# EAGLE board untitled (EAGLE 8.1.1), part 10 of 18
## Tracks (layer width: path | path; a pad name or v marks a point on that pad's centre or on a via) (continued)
S$9845 (continued)
  Bottom 0: 275.28,114.34 275.28,113.48
S$9846
  Bottom 0: 281.02,119.09 281.35,119.11
S$9847
  Bottom 0: 281.35,119.11 281.65,119.22
S$9848
  Bottom 0: 281.65,119.22 281.92,119.41
S$9849
  Bottom 0: 281.92,119.41 282.12,119.66
S$9850
  Bottom 0: 282.12,119.66 282.25,119.96
S$9851
  Bottom 0: 282.25,119.96 282.3,120.28
S$9852
  Bottom 0: 282.3,120.28 282.25,120.6
S$9853
  Bottom 0: 282.25,120.6 282.12,120.9
S$9854
  Bottom 0: 282.12,120.9 281.92,121.15
S$9855
  Bottom 0: 281.92,121.15 281.65,121.34
S$9856
  Bottom 0: 281.65,121.34 281.54,121.38
S$9857
  Bottom 0: 281.54,121.38 281.54,129.54
S$9858
  Bottom 0: 281.54,129.54 290.14,138.15
S$9859
  Bottom 0: 290.14,138.15 290.15,138.13
S$9860
  Bottom 0: 290.15,138.13 290.38,138.02
S$9861
  Bottom 0: 290.38,138.02 290.63,138
S$9862
  Bottom 0: 290.63,138 290.87,138.07
S$9863
  Bottom 0: 290.87,138.07 291.07,138.22
S$9864
  Bottom 0: 291.07,138.22 291.21,138.44
S$9865
  Bottom 0: 291.21,138.44 291.25,138.68
S$9866
  Bottom 0: 291.25,138.68 291.21,138.93
S$9867
  Bottom 0: 291.21,138.93 291.07,139.14
S$9868
  Bottom 0: 291.07,139.14 291,139.2
S$9869
  Bottom 0: 291,139.2 290.96,139.4
S$9870
  Bottom 0: 290.96,139.4 290.82,139.55
S$9871
  Bottom 0: 290.82,139.55 290.63,139.63
S$9872
  Bottom 0: 290.63,139.63 290.42,139.62
S$9873
  Bottom 0: 290.42,139.62 290.25,139.51
S$9874
  Bottom 0: 290.25,139.51 280.79,130.05
S$9875
  Bottom 0: 280.79,130.05 280.75,129.99
S$9876
  Bottom 0: 280.75,129.99 280.71,129.93
S$9877
  Bottom 0: 280.71,129.93 280.68,129.87
S$9878
  Bottom 0: 280.68,129.87 280.67,129.8
S$9879
  Bottom 0: 280.67,129.8 280.66,129.73
S$9880
  Bottom 0: 280.66,129.73 280.66,121.38
S$9881
  Bottom 0: 280.66,121.38 280.41,121.25
S$9882
  Bottom 0: 280.41,121.25 280.18,121.03
S$9883
  Bottom 0: 280.18,121.03 280,120.76
S$9884
  Bottom 0: 280,120.76 279.92,120.44
S$9885
  Bottom 0: 279.92,120.44 279.92,120.12
S$9886
  Bottom 0: 279.92,120.12 280,119.8
S$9887
  Bottom 0: 280,119.8 280.18,119.53
S$9888
  Bottom 0: 280.18,119.53 280.41,119.3
S$9889
  Bottom 0: 280.41,119.3 280.7,119.16
S$9890
  Bottom 0: 280.7,119.16 281.02,119.09
S$9891
  Bottom 0: 305.92,119.21 306.23,119.28
S$9892
  Bottom 0: 306.23,119.28 306.51,119.44
S$9893
  Bottom 0: 306.51,119.44 306.73,119.67
S$9894
  Bottom 0: 306.73,119.67 306.87,119.96
S$9895
  Bottom 0: 306.87,119.96 306.92,120.28
S$9896
  Bottom 0: 306.92,120.28 306.87,120.59
S$9897
  Bottom 0: 306.87,120.59 306.73,120.88
S$9898
  Bottom 0: 306.73,120.88 306.51,121.12
S$9899
  Bottom 0: 306.51,121.12 306.23,121.28
S$9900
  Bottom 0: 306.23,121.28 305.92,121.35
S$9901
  Bottom 0: 305.92,121.35 305.6,121.33
S$9902
  Bottom 0: 305.6,121.33 305.3,121.21
S$9903
  Bottom 0: 305.3,121.21 305.05,121.01
S$9904
  Bottom 0: 305.05,121.01 304.87,120.75
S$9905
  Bottom 0: 304.87,120.75 304.77,120.44
S$9906
  Bottom 0: 304.77,120.44 304.77,120.12
S$9907
  Bottom 0: 304.77,120.12 304.87,119.81
S$9908
  Bottom 0: 304.87,119.81 305.05,119.55
S$9909
  Bottom 0: 305.05,119.55 305.3,119.34
S$9910
  Bottom 0: 305.3,119.34 305.6,119.23
S$9911
  Bottom 0: 305.6,119.23 305.92,119.21
S$9912
  Bottom 0: 312.43,119.21 312.74,119.28
S$9913
  Bottom 0: 312.74,119.28 313.01,119.44
S$9914
  Bottom 0: 313.01,119.44 313.23,119.67
S$9915
  Bottom 0: 313.23,119.67 313.38,119.96
S$9916
  Bottom 0: 313.38,119.96 313.42,120.28
S$9917
  Bottom 0: 313.42,120.28 313.38,120.59
S$9918
  Bottom 0: 313.38,120.59 313.23,120.88
S$9919
  Bottom 0: 313.23,120.88 313.01,121.12
S$9920
  Bottom 0: 313.01,121.12 312.74,121.28
S$9921
  Bottom 0: 312.74,121.28 312.43,121.35
S$9922
  Bottom 0: 312.43,121.35 312.11,121.33
S$9923
  Bottom 0: 312.11,121.33 311.81,121.21
S$9924
  Bottom 0: 311.81,121.21 311.55,121.01
S$9925
  Bottom 0: 311.55,121.01 311.37,120.75
S$9926
  Bottom 0: 311.37,120.75 311.28,120.44
S$9927
  Bottom 0: 311.28,120.44 311.28,120.12
S$9928
  Bottom 0: 311.28,120.12 311.37,119.81
S$9929
  Bottom 0: 311.37,119.81 311.55,119.55
S$9930
  Bottom 0: 311.55,119.55 311.81,119.34
S$9931
  Bottom 0: 311.81,119.34 312.11,119.23
S$9932
  Bottom 0: 312.11,119.23 312.43,119.21
S$9933
  Bottom 0: 312.43,123.71 312.74,123.78
S$9934
  Bottom 0: 312.74,123.78 313.01,123.94
S$9935
  Bottom 0: 313.01,123.94 313.23,124.18
S$9936
  Bottom 0: 313.23,124.18 313.38,124.47
S$9937
  Bottom 0: 313.38,124.47 313.42,124.78
S$9938
  Bottom 0: 313.42,124.78 313.38,125.09
S$9939
  Bottom 0: 313.38,125.09 313.23,125.39
S$9940
  Bottom 0: 313.23,125.39 313.01,125.62
S$9941
  Bottom 0: 313.01,125.62 312.74,125.78
S$9942
  Bottom 0: 312.74,125.78 312.43,125.85
S$9943
  Bottom 0: 312.43,125.85 312.11,125.83
S$9944
  Bottom 0: 312.11,125.83 311.81,125.72
S$9945
  Bottom 0: 311.81,125.72 311.55,125.51
S$9946
  Bottom 0: 311.55,125.51 311.37,125.25
S$9947
  Bottom 0: 311.37,125.25 311.28,124.94
S$9948
  Bottom 0: 311.28,124.94 311.28,124.62
S$9949
  Bottom 0: 311.28,124.62 311.37,124.31
S$9950
  Bottom 0: 311.37,124.31 311.55,124.05
S$9951
  Bottom 0: 311.55,124.05 311.81,123.84
S$9952
  Bottom 0: 311.81,123.84 312.11,123.73
S$9953
  Bottom 0: 312.11,123.73 312.43,123.71
S$9954
  Bottom 0: 306.25,123.79 306.51,123.94
S$9955
  Bottom 0: 306.51,123.94 306.73,124.18
S$9956
  Bottom 0: 306.73,124.18 306.83,124.37
S$9957
  Bottom 0: 306.83,124.37 306.25,124.37
S$9958
  Bottom 0: 306.25,124.37 306.25,123.79
S$9959
  Bottom 0: 305.43,123.8 305.43,124.37
S$9960
  Bottom 0: 305.43,124.37 304.86,124.37
S$9961
  Bottom 0: 304.86,124.37 304.87,124.31
S$9962
  Bottom 0: 304.87,124.31 305.05,124.05
S$9963
  Bottom 0: 305.05,124.05 305.3,123.84
S$9964
  Bottom 0: 305.3,123.84 305.43,123.8
S$9965
  Bottom 0: 306.25,125.19 306.83,125.19
S$9966
  Bottom 0: 306.83,125.19 306.73,125.39
S$9967
  Bottom 0: 306.73,125.39 306.51,125.62
S$9968
  Bottom 0: 306.51,125.62 306.25,125.77
S$9969
  Bottom 0: 306.25,125.77 306.25,125.19
S$9970
  Bottom 0: 304.86,125.19 305.43,125.19
S$9971
  Bottom 0: 305.43,125.19 305.43,125.77
S$9972
  Bottom 0: 305.43,125.77 305.3,125.72
S$9973
  Bottom 0: 305.3,125.72 305.05,125.51
S$9974
  Bottom 0: 305.05,125.51 304.87,125.25
S$9975
  Bottom 0: 304.87,125.25 304.86,125.19
S$9976
  Bottom 0: 301.43,126.69 301.76,126.72
S$9977
  Bottom 0: 301.76,126.72 302.06,126.82
S$9978
  Bottom 0: 302.06,126.82 302.33,127.01
S$9979
  Bottom 0: 302.33,127.01 302.53,127.26
S$9980
  Bottom 0: 302.53,127.26 302.66,127.56
S$9981
  Bottom 0: 302.66,127.56 302.71,127.88
S$9982
  Bottom 0: 302.71,127.88 302.66,128.2
S$9983
  Bottom 0: 302.66,128.2 302.53,128.5
S$9984
  Bottom 0: 302.53,128.5 302.33,128.76
S$9985
  Bottom 0: 302.33,128.76 302.06,128.95
S$9986
  Bottom 0: 302.06,128.95 301.76,129.05
S$9987
  Bottom 0: 301.76,129.05 301.43,129.07
S$9988
  Bottom 0: 301.43,129.07 301.11,129.01
S$9989
  Bottom 0: 301.11,129.01 300.82,128.86
S$9990
  Bottom 0: 300.82,128.86 300.59,128.64
S$9991
  Bottom 0: 300.59,128.64 300.42,128.36
S$9992
  Bottom 0: 300.42,128.36 300.33,128.05
S$9993
  Bottom 0: 300.33,128.05 300.33,127.72
S$9994
  Bottom 0: 300.33,127.72 300.42,127.41
S$9995
  Bottom 0: 300.42,127.41 300.59,127.13
S$9996
  Bottom 0: 300.59,127.13 300.82,126.91
S$9997
  Bottom 0: 300.82,126.91 301.11,126.76
S$9998
  Bottom 0: 301.11,126.76 301.43,126.69
S$9999
  Bottom 0: 303.97,126.69 304.3,126.72
S$10000
  Bottom 0: 304.3,126.72 304.6,126.82
S$10001
  Bottom 0: 304.6,126.82 304.87,127.01
S$10002
  Bottom 0: 304.87,127.01 305.07,127.26
S$10003
  Bottom 0: 305.07,127.26 305.2,127.56
S$10004
  Bottom 0: 305.2,127.56 305.25,127.88
S$10005
  Bottom 0: 305.25,127.88 305.2,128.2
S$10006
  Bottom 0: 305.2,128.2 305.07,128.5
S$10007
  Bottom 0: 305.07,128.5 304.87,128.76
S$10008
  Bottom 0: 304.87,128.76 304.6,128.95
S$10009
  Bottom 0: 304.6,128.95 304.3,129.05
S$10010
  Bottom 0: 304.3,129.05 303.97,129.07
S$10011
  Bottom 0: 303.97,129.07 303.65,129.01
S$10012
  Bottom 0: 303.65,129.01 303.36,128.86
S$10013
  Bottom 0: 303.36,128.86 303.13,128.64
S$10014
  Bottom 0: 303.13,128.64 302.96,128.36
S$10015
  Bottom 0: 302.96,128.36 302.87,128.05
S$10016
  Bottom 0: 302.87,128.05 302.87,127.72
S$10017
  Bottom 0: 302.87,127.72 302.96,127.41
S$10018
  Bottom 0: 302.96,127.41 303.13,127.13
S$10019
  Bottom 0: 303.13,127.13 303.36,126.91
S$10020
  Bottom 0: 303.36,126.91 303.65,126.76
S$10021
  Bottom 0: 303.65,126.76 303.97,126.69
S$10022
  Bottom 0: 309.05,126.69 309.38,126.72
S$10023
  Bottom 0: 309.38,126.72 309.68,126.82
S$10024
  Bottom 0: 309.68,126.82 309.95,127.01
S$10025
  Bottom 0: 309.95,127.01 310.15,127.26
S$10026
  Bottom 0: 310.15,127.26 310.28,127.56
S$10027
  Bottom 0: 310.28,127.56 310.33,127.88
S$10028
  Bottom 0: 310.33,127.88 310.28,128.2
S$10029
  Bottom 0: 310.28,128.2 310.15,128.5
S$10030
  Bottom 0: 310.15,128.5 309.95,128.76
S$10031
  Bottom 0: 309.95,128.76 309.68,128.95
S$10032
  Bottom 0: 309.68,128.95 309.38,129.05
S$10033
  Bottom 0: 309.38,129.05 309.05,129.07
S$10034
  Bottom 0: 309.05,129.07 308.73,129.01
S$10035
  Bottom 0: 308.73,129.01 308.44,128.86
S$10036
  Bottom 0: 308.44,128.86 308.21,128.64
S$10037
  Bottom 0: 308.21,128.64 308.04,128.36
S$10038
  Bottom 0: 308.04,128.36 307.95,128.05
S$10039
  Bottom 0: 307.95,128.05 307.95,127.72
S$10040
  Bottom 0: 307.95,127.72 308.04,127.41
S$10041
  Bottom 0: 308.04,127.41 308.21,127.13
S$10042
  Bottom 0: 308.21,127.13 308.44,126.91
S$10043
  Bottom 0: 308.44,126.91 308.73,126.76
S$10044
  Bottom 0: 308.73,126.76 309.05,126.69
S$10045
  Bottom 0: 289.28,126.79 289.36,126.82
S$10046
  Bottom 0: 289.36,126.82 289.63,127.01
S$10047
  Bottom 0: 289.63,127.01 289.83,127.26
S$10048
  Bottom 0: 289.83,127.26 289.9,127.42
S$10049
  Bottom 0: 289.9,127.42 289.28,127.42
S$10050
  Bottom 0: 289.28,127.42 289.28,126.79
S$10051
  Bottom 0: 288.35,126.8 288.35,127.42
S$10052
  Bottom 0: 288.35,127.42 287.71,127.42
S$10053
  Bottom 0: 287.71,127.42 287.72,127.41
S$10054
  Bottom 0: 287.72,127.41 287.89,127.13
S$10055
  Bottom 0: 287.89,127.13 288.12,126.91
S$10056
  Bottom 0: 288.12,126.91 288.35,126.8
S$10057
  Bottom 0: 289.28,128.35 289.9,128.35
S$10058
  Bottom 0: 289.9,128.35 289.83,128.5
S$10059
  Bottom 0: 289.83,128.5 289.63,128.76
S$10060
  Bottom 0: 289.63,128.76 289.36,128.95
S$10061
  Bottom 0: 289.36,128.95 289.28,128.98
S$10062
  Bottom 0: 289.28,128.98 289.28,128.35
S$10063
  Bottom 0: 287.71,128.35 288.35,128.35
S$10064
  Bottom 0: 288.35,128.35 288.35,128.97
S$10065
  Bottom 0: 288.35,128.97 288.12,128.86
S$10066
  Bottom 0: 288.12,128.86 287.89,128.64
S$10067
  Bottom 0: 287.89,128.64 287.72,128.36
S$10068
  Bottom 0: 287.72,128.36 287.71,128.35
S$10069
  Bottom 0: 292.49,130.78 292.73,130.85
S$10070
  Bottom 0: 292.73,130.85 292.93,131
S$10071
  Bottom 0: 292.93,131 293.06,131.21
S$10072
  Bottom 0: 293.06,131.21 293.11,131.46
S$10073
  Bottom 0: 293.11,131.46 293.06,131.71
S$10074
  Bottom 0: 293.06,131.71 292.93,131.92
S$10075
  Bottom 0: 292.93,131.92 292.86,131.97
S$10076
  Bottom 0: 292.86,131.97 292.86,133.85
S$10077
  Bottom 0: 292.86,133.85 301.05,142.03
S$10078
  Bottom 0: 301.05,142.03 301.11,142
S$10079
  Bottom 0: 301.11,142 301.43,141.93
S$10080
  Bottom 0: 301.43,141.93 301.76,141.96
S$10081
  Bottom 0: 301.76,141.96 302.06,142.06
S$10082
  Bottom 0: 302.06,142.06 302.33,142.25
S$10083
  Bottom 0: 302.33,142.25 302.53,142.5
S$10084
  Bottom 0: 302.53,142.5 302.66,142.8
S$10085
  Bottom 0: 302.66,142.8 302.71,143.12
S$10086
  Bottom 0: 302.71,143.12 302.66,143.44
S$10087
  Bottom 0: 302.66,143.44 302.53,143.74
S$10088
  Bottom 0: 302.53,143.74 302.33,144
S$10089
  Bottom 0: 302.33,144 302.06,144.19
S$10090
  Bottom 0: 302.06,144.19 301.76,144.29
S$10091
  Bottom 0: 301.76,144.29 301.43,144.31
S$10092
  Bottom 0: 301.43,144.31 301.11,144.25
S$10093
  Bottom 0: 301.11,144.25 300.82,144.1
S$10094
  Bottom 0: 300.82,144.1 300.59,143.88
S$10095
  Bottom 0: 300.59,143.88 300.42,143.6
S$10096
  Bottom 0: 300.42,143.6 300.33,143.29
S$10097
  Bottom 0: 300.33,143.29 300.33,142.96
S$10098
  Bottom 0: 300.33,142.96 300.42,142.66
S$10099
  Bottom 0: 300.42,142.66 292.11,134.35
S$10100
  Bottom 0: 292.11,134.35 292.02,134.24
S$10101
  Bottom 0: 292.02,134.24 292,134.17
S$10102
  Bottom 0: 292,134.17 291.98,134.11
S$10103
  Bottom 0: 291.98,134.11 291.98,134.04
S$10104
  Bottom 0: 291.98,134.04 291.98,131.97
S$10105
  Bottom 0: 291.98,131.97 291.84,131.82
S$10106
  Bottom 0: 291.84,131.82 291.75,131.59
S$10107
  Bottom 0: 291.75,131.59 291.75,131.33
S$10108
  Bottom 0: 291.75,131.33 291.84,131.1
S$10109
  Bottom 0: 291.84,131.1 292.01,130.91
S$10110
  Bottom 0: 292.01,130.91 292.24,130.8
S$10111
  Bottom 0: 292.24,130.8 292.49,130.78
S$10112
  Bottom 0: 311.59,141.93 311.92,141.96
S$10113
  Bottom 0: 311.92,141.96 312.22,142.06
S$10114
  Bottom 0: 312.22,142.06 312.49,142.25
S$10115
  Bottom 0: 312.49,142.25 312.69,142.5
S$10116
  Bottom 0: 312.69,142.5 312.82,142.8
S$10117
  Bottom 0: 312.82,142.8 312.87,143.12
S$10118
  Bottom 0: 312.87,143.12 312.82,143.44
S$10119
  Bottom 0: 312.82,143.44 312.69,143.74
S$10120
  Bottom 0: 312.69,143.74 312.49,144
S$10121
  Bottom 0: 312.49,144 312.22,144.19
S$10122
  Bottom 0: 312.22,144.19 311.92,144.29
S$10123
  Bottom 0: 311.92,144.29 311.59,144.31
S$10124
  Bottom 0: 311.59,144.31 311.27,144.25
S$10125
  Bottom 0: 311.27,144.25 310.98,144.1
S$10126
  Bottom 0: 310.98,144.1 310.75,143.88
S$10127
  Bottom 0: 310.75,143.88 310.58,143.6
S$10128
  Bottom 0: 310.58,143.6 310.49,143.29
S$10129
  Bottom 0: 310.49,143.29 310.49,142.96
S$10130
  Bottom 0: 310.49,142.96 310.58,142.65
S$10131
  Bottom 0: 310.58,142.65 310.75,142.37
S$10132
  Bottom 0: 310.75,142.37 310.98,142.15
S$10133
  Bottom 0: 310.98,142.15 311.27,142
S$10134
  Bottom 0: 311.27,142 311.59,141.93
S$10135
  Bottom 0: 309.05,141.93 309.38,141.96
S$10136
  Bottom 0: 309.38,141.96 309.68,142.06
S$10137
  Bottom 0: 309.68,142.06 309.95,142.25
S$10138
  Bottom 0: 309.95,142.25 310.15,142.5
S$10139
  Bottom 0: 310.15,142.5 310.28,142.8
S$10140
  Bottom 0: 310.28,142.8 310.33,143.12
S$10141
  Bottom 0: 310.33,143.12 310.28,143.44
S$10142
  Bottom 0: 310.28,143.44 310.15,143.74
S$10143
  Bottom 0: 310.15,143.74 309.95,144
S$10144
  Bottom 0: 309.95,144 309.68,144.19
S$10145
  Bottom 0: 309.68,144.19 309.38,144.29
S$10146
  Bottom 0: 309.38,144.29 309.05,144.31
S$10147
  Bottom 0: 309.05,144.31 308.73,144.25
S$10148
  Bottom 0: 308.73,144.25 308.44,144.1
S$10149
  Bottom 0: 308.44,144.1 308.21,143.88
S$10150
  Bottom 0: 308.21,143.88 308.04,143.6
S$10151
  Bottom 0: 308.04,143.6 307.95,143.29
S$10152
  Bottom 0: 307.95,143.29 307.95,142.96
S$10153
  Bottom 0: 307.95,142.96 308.04,142.65
S$10154
  Bottom 0: 308.04,142.65 308.21,142.37
S$10155
  Bottom 0: 308.21,142.37 308.44,142.15
S$10156
  Bottom 0: 308.44,142.15 308.73,142
S$10157
  Bottom 0: 308.73,142 309.05,141.93
S$10158
  Bottom 0: 298.89,141.93 299.22,141.96
S$10159
  Bottom 0: 299.22,141.96 299.52,142.06
S$10160
  Bottom 0: 299.52,142.06 299.79,142.25
S$10161
  Bottom 0: 299.79,142.25 299.99,142.5
S$10162
  Bottom 0: 299.99,142.5 300.12,142.8
S$10163
  Bottom 0: 300.12,142.8 300.17,143.12
S$10164
  Bottom 0: 300.17,143.12 300.12,143.44
S$10165
  Bottom 0: 300.12,143.44 300.06,143.58
S$10166
  Bottom 0: 300.06,143.58 301.1,144.63
S$10167
  Bottom 0: 301.1,144.63 301.14,144.68
S$10168
  Bottom 0: 301.14,144.68 301.18,144.74
S$10169
  Bottom 0: 301.18,144.74 301.2,144.8
S$10170
  Bottom 0: 301.2,144.8 301.22,144.86
S$10171
  Bottom 0: 301.22,144.86 301.22,144.94
S$10172
  Bottom 0: 301.22,144.94 301.22,150.65
S$10173
  Bottom 0: 301.22,150.65 301.28,150.63
S$10174
  Bottom 0: 301.28,150.63 301.63,150.61
S$10175
  Bottom 0: 301.63,150.61 301.98,150.67
S$10176
  Bottom 0: 301.98,150.67 302.29,150.82
S$10177
  Bottom 0: 302.29,150.82 302.56,151.05
S$10178
  Bottom 0: 302.56,151.05 302.77,151.33
S$10179
  Bottom 0: 302.77,151.33 302.89,151.66
S$10180
  Bottom 0: 302.89,151.66 302.94,152
S$10181
  Bottom 0: 302.94,152 302.89,152.35
S$10182
  Bottom 0: 302.89,152.35 302.77,152.67
S$10183
  Bottom 0: 302.77,152.67 302.56,152.96
S$10184
  Bottom 0: 302.56,152.96 302.29,153.18
S$10185
  Bottom 0: 302.29,153.18 301.98,153.34
S$10186
  Bottom 0: 301.98,153.34 301.63,153.39
S$10187
  Bottom 0: 301.63,153.39 301.28,153.38
S$10188
  Bottom 0: 301.28,153.38 301.17,153.34
S$10189
  Bottom 0: 301.17,153.34 300.87,153.39
S$10190
  Bottom 0: 300.87,153.39 300.52,153.38
S$10191
  Bottom 0: 300.52,153.38 300.19,153.27
S$10192
  Bottom 0: 300.19,153.27 299.89,153.08
S$10193
  Bottom 0: 299.89,153.08 299.65,152.83
S$10194
  Bottom 0: 299.65,152.83 299.48,152.52
S$10195
  Bottom 0: 299.48,152.52 299.39,152.18
S$10196
  Bottom 0: 299.39,152.18 299.39,151.83
S$10197
  Bottom 0: 299.39,151.83 299.48,151.49
S$10198
  Bottom 0: 299.48,151.49 299.65,151.18
S$10199
  Bottom 0: 299.65,151.18 299.89,150.93
S$10200
  Bottom 0: 299.89,150.93 300.19,150.74
S$10201
  Bottom 0: 300.19,150.74 300.34,150.69
S$10202
  Bottom 0: 300.34,150.69 300.34,145.12
S$10203
  Bottom 0: 300.34,145.12 299.44,144.22
S$10204
  Bottom 0: 299.44,144.22 299.22,144.29
S$10205
  Bottom 0: 299.22,144.29 298.89,144.31
S$10206
  Bottom 0: 298.89,144.31 298.57,144.25
S$10207
  Bottom 0: 298.57,144.25 298.28,144.1
S$10208
  Bottom 0: 298.28,144.1 298.05,143.88
S$10209
  Bottom 0: 298.05,143.88 297.88,143.6
S$10210
  Bottom 0: 297.88,143.6 297.79,143.29
S$10211
  Bottom 0: 297.79,143.29 297.79,142.96
S$10212
  Bottom 0: 297.79,142.96 297.88,142.65
S$10213
  Bottom 0: 297.88,142.65 298.05,142.37
S$10214
  Bottom 0: 298.05,142.37 298.28,142.15
S$10215
  Bottom 0: 298.28,142.15 298.57,142
S$10216
  Bottom 0: 298.57,142 298.89,141.93
S$10217
  Bottom 0: 296.35,141.93 296.68,141.96
S$10218
  Bottom 0: 296.68,141.96 296.98,142.06
S$10219
  Bottom 0: 296.98,142.06 297.25,142.25
S$10220
  Bottom 0: 297.25,142.25 297.45,142.5
S$10221
  Bottom 0: 297.45,142.5 297.58,142.8
S$10222
  Bottom 0: 297.58,142.8 297.63,143.12
S$10223
  Bottom 0: 297.63,143.12 297.58,143.44
S$10224
  Bottom 0: 297.58,143.44 297.45,143.74
S$10225
  Bottom 0: 297.45,143.74 297.25,144
S$10226
  Bottom 0: 297.25,144 296.98,144.19
S$10227
  Bottom 0: 296.98,144.19 296.68,144.29
S$10228
  Bottom 0: 296.68,144.29 296.35,144.31
S$10229
  Bottom 0: 296.35,144.31 296.03,144.25
S$10230
  Bottom 0: 296.03,144.25 295.74,144.1
S$10231
  Bottom 0: 295.74,144.1 295.51,143.88
S$10232
  Bottom 0: 295.51,143.88 295.34,143.6
S$10233
  Bottom 0: 295.34,143.6 295.25,143.29
S$10234
  Bottom 0: 295.25,143.29 295.25,142.96
S$10235
  Bottom 0: 295.25,142.96 295.34,142.65
S$10236
  Bottom 0: 295.34,142.65 295.51,142.37
S$10237
  Bottom 0: 295.51,142.37 295.74,142.15
S$10238
  Bottom 0: 295.74,142.15 296.03,142
S$10239
  Bottom 0: 296.03,142 296.35,141.93
S$10240
  Bottom 0: 288.73,141.93 289.06,141.96
S$10241
  Bottom 0: 289.06,141.96 289.36,142.06
S$10242
  Bottom 0: 289.36,142.06 289.63,142.25
S$10243
  Bottom 0: 289.63,142.25 289.83,142.5
S$10244
  Bottom 0: 289.83,142.5 289.96,142.8
S$10245
  Bottom 0: 289.96,142.8 290.01,143.12
S$10246
  Bottom 0: 290.01,143.12 289.96,143.44
S$10247
  Bottom 0: 289.96,143.44 289.83,143.74
S$10248
  Bottom 0: 289.83,143.74 289.63,144
S$10249
  Bottom 0: 289.63,144 289.36,144.19
S$10250
  Bottom 0: 289.36,144.19 289.06,144.29
S$10251
  Bottom 0: 289.06,144.29 288.73,144.31
S$10252
  Bottom 0: 288.73,144.31 288.41,144.25
S$10253
  Bottom 0: 288.41,144.25 288.12,144.1
S$10254
  Bottom 0: 288.12,144.1 287.89,143.88
S$10255
  Bottom 0: 287.89,143.88 287.72,143.6
S$10256
  Bottom 0: 287.72,143.6 287.63,143.29
S$10257
  Bottom 0: 287.63,143.29 287.63,142.96
S$10258
  Bottom 0: 287.63,142.96 287.72,142.65
S$10259
  Bottom 0: 287.72,142.65 287.89,142.37
S$10260
  Bottom 0: 287.89,142.37 288.12,142.15
S$10261
  Bottom 0: 288.12,142.15 288.41,142
S$10262
  Bottom 0: 288.41,142 288.73,141.93
S$10263
  Bottom 0: 286.19,141.93 286.52,141.96
S$10264
  Bottom 0: 286.52,141.96 286.82,142.06
S$10265
  Bottom 0: 286.82,142.06 287.09,142.25
S$10266
  Bottom 0: 287.09,142.25 287.29,142.5
S$10267
  Bottom 0: 287.29,142.5 287.42,142.8
S$10268
  Bottom 0: 287.42,142.8 287.47,143.12
S$10269
  Bottom 0: 287.47,143.12 287.42,143.44
S$10270
  Bottom 0: 287.42,143.44 287.29,143.74
S$10271
  Bottom 0: 287.29,143.74 287.09,144
S$10272
  Bottom 0: 287.09,144 286.82,144.19
S$10273
  Bottom 0: 286.82,144.19 286.52,144.29
S$10274
  Bottom 0: 286.52,144.29 286.19,144.31
S$10275
  Bottom 0: 286.19,144.31 285.87,144.25
S$10276
  Bottom 0: 285.87,144.25 285.58,144.1
S$10277
  Bottom 0: 285.58,144.1 285.35,143.88
S$10278
  Bottom 0: 285.35,143.88 285.18,143.6
S$10279
  Bottom 0: 285.18,143.6 285.09,143.29
S$10280
  Bottom 0: 285.09,143.29 285.09,142.96
S$10281
  Bottom 0: 285.09,142.96 285.18,142.65
S$10282
  Bottom 0: 285.18,142.65 285.35,142.37
S$10283
  Bottom 0: 285.35,142.37 285.58,142.15
S$10284
  Bottom 0: 285.58,142.15 285.87,142
S$10285
  Bottom 0: 285.87,142 286.19,141.93
S$10286
  Bottom 0: 294.36,142.03 294.44,142.06
S$10287
  Bottom 0: 294.44,142.06 294.71,142.25
S$10288
  Bottom 0: 294.71,142.25 294.91,142.5
S$10289
  Bottom 0: 294.91,142.5 294.98,142.66
S$10290
  Bottom 0: 294.98,142.66 294.36,142.66
S$10291
  Bottom 0: 294.36,142.66 294.36,142.03
S$10292
  Bottom 0: 291.82,142.03 291.9,142.06
S$10293
  Bottom 0: 291.9,142.06 292.17,142.25
S$10294
  Bottom 0: 292.17,142.25 292.37,142.5
S$10295
  Bottom 0: 292.37,142.5 292.44,142.66
S$10296
  Bottom 0: 292.44,142.66 291.82,142.66
S$10297
  Bottom 0: 291.82,142.66 291.82,142.03
S$10298
  Bottom 0: 293.43,142.04 293.43,142.66
S$10299
  Bottom 0: 293.43,142.66 292.79,142.66
S$10300
  Bottom 0: 292.79,142.66 292.8,142.65
S$10301
  Bottom 0: 292.8,142.65 292.97,142.37
S$10302
  Bottom 0: 292.97,142.37 293.2,142.15
S$10303
  Bottom 0: 293.2,142.15 293.43,142.04
S$10304
  Bottom 0: 290.89,142.04 290.89,142.66
S$10305
  Bottom 0: 290.89,142.66 290.25,142.66
S$10306
  Bottom 0: 290.25,142.66 290.26,142.65
S$10307
  Bottom 0: 290.26,142.65 290.43,142.37
S$10308
  Bottom 0: 290.43,142.37 290.66,142.15
S$10309
  Bottom 0: 290.66,142.15 290.89,142.04
S$10310
  Bottom 0: 294.36,143.59 294.98,143.59
S$10311
  Bottom 0: 294.98,143.59 294.91,143.74
S$10312
  Bottom 0: 294.91,143.74 294.71,144
S$10313
  Bottom 0: 294.71,144 294.44,144.19
S$10314
  Bottom 0: 294.44,144.19 294.36,144.22
S$10315
  Bottom 0: 294.36,144.22 294.36,143.59
S$10316
  Bottom 0: 292.79,143.59 293.43,143.59
S$10317
  Bottom 0: 293.43,143.59 293.43,144.21
S$10318
  Bottom 0: 293.43,144.21 293.2,144.1
S$10319
  Bottom 0: 293.2,144.1 292.97,143.88
S$10320
  Bottom 0: 292.97,143.88 292.8,143.6
S$10321
  Bottom 0: 292.8,143.6 292.79,143.59
S$10322
  Bottom 0: 291.82,143.59 292.44,143.59
S$10323
  Bottom 0: 292.44,143.59 292.37,143.74
S$10324
  Bottom 0: 292.37,143.74 292.17,144
S$10325
  Bottom 0: 292.17,144 291.9,144.19
S$10326
  Bottom 0: 291.9,144.19 291.82,144.22
S$10327
  Bottom 0: 291.82,144.22 291.82,143.59
S$10328
  Bottom 0: 290.25,143.59 290.89,143.59
S$10329
  Bottom 0: 290.89,143.59 290.89,144.21
S$10330
  Bottom 0: 290.89,144.21 290.66,144.1
S$10331
  Bottom 0: 290.66,144.1 290.43,143.88
S$10332
  Bottom 0: 290.43,143.88 290.26,143.6
S$10333
  Bottom 0: 290.26,143.6 290.25,143.59
S$10334
  Bottom 0: 294.52,148.07 294.82,148.13
S$10335
  Bottom 0: 294.82,148.13 294.93,148.09
S$10336
  Bottom 0: 294.93,148.09 295.28,148.07
S$10337
  Bottom 0: 295.28,148.07 295.63,148.13
S$10338
  Bottom 0: 295.63,148.13 295.94,148.28
S$10339
  Bottom 0: 295.94,148.28 296.21,148.51
S$10340
  Bottom 0: 296.21,148.51 296.42,148.79
S$10341
  Bottom 0: 296.42,148.79 296.55,149.12
S$10342
  Bottom 0: 296.55,149.12 296.59,149.46
S$10343
  Bottom 0: 296.59,149.46 296.55,149.81
S$10344
  Bottom 0: 296.55,149.81 296.42,150.13
S$10345
  Bottom 0: 296.42,150.13 296.21,150.42
S$10346
  Bottom 0: 296.21,150.42 295.94,150.64
S$10347
  Bottom 0: 295.94,150.64 295.63,150.79
S$10348
  Bottom 0: 295.63,150.79 295.28,150.85
S$10349
  Bottom 0: 295.28,150.85 294.93,150.84
S$10350
  Bottom 0: 294.93,150.84 294.82,150.8
S$10351
  Bottom 0: 294.82,150.8 294.52,150.85
S$10352
  Bottom 0: 294.52,150.85 294.17,150.84
S$10353
  Bottom 0: 294.17,150.84 293.83,150.73
S$10354
  Bottom 0: 293.83,150.73 293.54,150.54
S$10355
  Bottom 0: 293.54,150.54 293.3,150.29
S$10356
  Bottom 0: 293.3,150.29 293.13,149.98
S$10357
  Bottom 0: 293.13,149.98 293.11,149.91
S$10358
  Bottom 0: 293.11,149.91 289.96,149.91
S$10359
  Bottom 0: 289.96,149.91 289.21,150.66
S$10360
  Bottom 0: 289.21,150.66 289.23,150.68
S$10361
  Bottom 0: 289.23,150.68 289.27,150.98
S$10362
  Bottom 0: 289.27,150.98 289.23,151.28
S$10363
  Bottom 0: 289.23,151.28 289.09,151.56
S$10364
  Bottom 0: 289.09,151.56 288.89,151.78
S$10365
  Bottom 0: 288.89,151.78 288.62,151.93
S$10366
  Bottom 0: 288.62,151.93 288.33,151.99
S$10367
  Bottom 0: 288.33,151.99 288.03,151.97
S$10368
  Bottom 0: 288.03,151.97 287.74,151.86
S$10369
  Bottom 0: 287.74,151.86 287.51,151.67
S$10370
  Bottom 0: 287.51,151.67 287.34,151.43
S$10371
  Bottom 0: 287.34,151.43 287.25,151.13
S$10372
  Bottom 0: 287.25,151.13 287.25,150.83
S$10373
  Bottom 0: 287.25,150.83 287.34,150.54
S$10374
  Bottom 0: 287.34,150.54 287.51,150.29
S$10375
  Bottom 0: 287.51,150.29 287.74,150.1
S$10376
  Bottom 0: 287.74,150.1 288.03,149.99
S$10377
  Bottom 0: 288.03,149.99 288.33,149.97
S$10378
  Bottom 0: 288.33,149.97 288.58,150.03
S$10379
  Bottom 0: 288.58,150.03 289.46,149.15
S$10380
  Bottom 0: 289.46,149.15 289.51,149.11
S$10381
  Bottom 0: 289.51,149.11 289.57,149.07
S$10382
  Bottom 0: 289.57,149.07 289.64,149.04
S$10383
  Bottom 0: 289.64,149.04 289.7,149.03
S$10384
  Bottom 0: 289.7,149.03 289.77,149.02
S$10385
  Bottom 0: 289.77,149.02 293.11,149.02
S$10386
  Bottom 0: 293.11,149.02 293.13,148.95
S$10387
  Bottom 0: 293.13,148.95 293.3,148.64
S$10388
  Bottom 0: 293.3,148.64 293.54,148.39
S$10389
  Bottom 0: 293.54,148.39 293.83,148.2
S$10390
  Bottom 0: 293.83,148.2 294.17,148.09
S$10391
  Bottom 0: 294.17,148.09 294.52,148.07
S$10392
  Bottom 0: 296.97,152.26 297.35,152.3
S$10393
  Bottom 0: 297.35,152.3 297.73,152.26
S$10394
  Bottom 0: 297.73,152.26 298.18,152.3
S$10395
  Bottom 0: 298.18,152.3 298.61,152.43
S$10396
  Bottom 0: 298.61,152.43 299,152.64
S$10397
  Bottom 0: 299,152.64 299.35,152.93
S$10398
  Bottom 0: 299.35,152.93 299.63,153.27
S$10399
  Bottom 0: 299.63,153.27 299.85,153.67
S$10400
  Bottom 0: 299.85,153.67 299.97,154.1
S$10401
  Bottom 0: 299.97,154.1 300.02,154.54
S$10402
  Bottom 0: 300.02,154.54 299.97,154.99
S$10403
  Bottom 0: 299.97,154.99 299.85,155.42
S$10404
  Bottom 0: 299.85,155.42 299.63,155.81
S$10405
  Bottom 0: 299.63,155.81 299.35,156.16
S$10406
  Bottom 0: 299.35,156.16 299,156.44
S$10407
  Bottom 0: 299,156.44 298.61,156.66
S$10408
  Bottom 0: 298.61,156.66 298.18,156.78
S$10409
  Bottom 0: 298.18,156.78 297.73,156.83
S$10410
  Bottom 0: 297.73,156.83 297.35,156.79
S$10411
  Bottom 0: 297.35,156.79 296.97,156.83
S$10412
  Bottom 0: 296.97,156.83 296.52,156.78
S$10413
  Bottom 0: 296.52,156.78 296.1,156.66
S$10414
  Bottom 0: 296.1,156.66 295.7,156.44
S$10415
  Bottom 0: 295.7,156.44 295.36,156.16
S$10416
  Bottom 0: 295.36,156.16 295.07,155.81
S$10417
  Bottom 0: 295.07,155.81 294.86,155.42
S$10418
  Bottom 0: 294.86,155.42 294.73,154.99
S$10419
  Bottom 0: 294.73,154.99 294.69,154.54
S$10420
  Bottom 0: 294.69,154.54 294.73,154.1
S$10421
  Bottom 0: 294.73,154.1 294.86,153.67
S$10422
  Bottom 0: 294.86,153.67 295.07,153.27
S$10423
  Bottom 0: 295.07,153.27 295.36,152.93
S$10424
  Bottom 0: 295.36,152.93 295.7,152.64
S$10425
  Bottom 0: 295.7,152.64 296.1,152.43
S$10426
  Bottom 0: 296.1,152.43 296.52,152.3
S$10427
  Bottom 0: 296.52,152.3 296.97,152.26
S$10428
  Bottom 0: 288.33,157.59 288.62,157.66
S$10429
  Bottom 0: 288.62,157.66 288.89,157.81
S$10430
  Bottom 0: 288.89,157.81 289.09,158.03
S$10431
  Bottom 0: 289.09,158.03 289.23,158.3
S$10432
  Bottom 0: 289.23,158.3 289.27,158.6
S$10433
  Bottom 0: 289.27,158.6 289.23,158.9
S$10434
  Bottom 0: 289.23,158.9 289.09,159.18
S$10435
  Bottom 0: 289.09,159.18 288.89,159.4
S$10436
  Bottom 0: 288.89,159.4 288.62,159.55
S$10437
  Bottom 0: 288.62,159.55 288.33,159.61
S$10438
  Bottom 0: 288.33,159.61 288.03,159.59
S$10439
  Bottom 0: 288.03,159.59 287.74,159.48
S$10440
  Bottom 0: 287.74,159.48 287.51,159.29
S$10441
  Bottom 0: 287.51,159.29 287.34,159.04
S$10442
  Bottom 0: 287.34,159.04 287.25,158.75
S$10443
  Bottom 0: 287.25,158.75 287.25,158.45
S$10444
  Bottom 0: 287.25,158.45 287.34,158.16
S$10445
  Bottom 0: 287.34,158.16 287.51,157.91
S$10446
  Bottom 0: 287.51,157.91 287.74,157.72
S$10447
  Bottom 0: 287.74,157.72 288.03,157.61
S$10448
  Bottom 0: 288.03,157.61 288.33,157.59
S$10449
  Bottom 0: 284,163.83 284.54,163.83
S$10450
  Bottom 0: 284.54,163.83 284.62,163.84
S$10451
  Bottom 0: 284.62,163.84 284.69,163.88
S$10452
  Bottom 0: 284.69,163.88 284.74,163.93
S$10453
  Bottom 0: 284.74,163.93 284.79,164.01
S$10454
  Bottom 0: 284.79,164.01 284.8,164.08
S$10455
  Bottom 0: 284.8,164.08 284.8,164.38
S$10456
  Bottom 0: 284.8,164.38 284,164.38
S$10457
  Bottom 0: 284,164.38 284,163.83
S$10458
  Bottom 0: 282.38,163.83 282.93,163.83
S$10459
  Bottom 0: 282.93,163.83 282.93,164.38
S$10460
  Bottom 0: 282.93,164.38 282.13,164.38
S$10461
  Bottom 0: 282.13,164.38 282.13,164.08
S$10462
  Bottom 0: 282.13,164.08 282.14,164.01
S$10463
  Bottom 0: 282.14,164.01 282.18,163.93
S$10464
  Bottom 0: 282.18,163.93 282.24,163.88
S$10465
  Bottom 0: 282.24,163.88 282.31,163.84
S$10466
  Bottom 0: 282.31,163.84 282.38,163.83
S$10467
  Bottom 0: 284,164.98 284.8,164.98
S$10468
  Bottom 0: 284.8,164.98 284.8,165.28
S$10469
  Bottom 0: 284.8,165.28 284.79,165.36
S$10470
  Bottom 0: 284.79,165.36 284.74,165.43
S$10471
  Bottom 0: 284.74,165.43 284.69,165.49
S$10472
  Bottom 0: 284.69,165.49 284.62,165.53
S$10473
  Bottom 0: 284.62,165.53 284.54,165.54
S$10474
  Bottom 0: 284.54,165.54 284,165.54
S$10475
  Bottom 0: 284,165.54 284,164.98
S$10476
  Bottom 0: 282.13,164.98 282.93,164.98
S$10477
  Bottom 0: 282.93,164.98 282.93,165.54
S$10478
  Bottom 0: 282.93,165.54 282.38,165.54
S$10479
  Bottom 0: 282.38,165.54 282.31,165.53
S$10480
  Bottom 0: 282.31,165.53 282.24,165.49
S$10481
  Bottom 0: 282.24,165.49 282.18,165.43
S$10482
  Bottom 0: 282.18,165.43 282.14,165.36
S$10483
  Bottom 0: 282.14,165.36 282.13,165.28
S$10484
  Bottom 0: 282.13,165.28 282.13,164.98
S$10485
  Bottom 0: 306.27,168.1 306.79,168.1
S$10486
  Bottom 0: 306.79,168.1 307.3,168.19
S$10487
  Bottom 0: 307.3,168.19 307.79,168.36
S$10488
  Bottom 0: 307.79,168.36 308.24,168.6
S$10489
  Bottom 0: 308.24,168.6 308.66,168.92
S$10490
  Bottom 0: 308.66,168.92 309.01,169.3
S$10491
  Bottom 0: 309.01,169.3 309.29,169.73
S$10492
  Bottom 0: 309.29,169.73 309.5,170.21
S$10493
  Bottom 0: 309.5,170.21 309.63,170.71
S$10494
  Bottom 0: 309.63,170.71 309.67,171.23
S$10495
  Bottom 0: 309.67,171.23 309.63,171.75
S$10496
  Bottom 0: 309.63,171.75 309.5,172.24
S$10497
  Bottom 0: 309.5,172.24 309.29,172.72
S$10498
  Bottom 0: 309.29,172.72 309.01,173.15
S$10499
  Bottom 0: 309.01,173.15 308.66,173.53
S$10500
  Bottom 0: 308.66,173.53 308.24,173.85
S$10501
  Bottom 0: 308.24,173.85 307.79,174.1
S$10502
  Bottom 0: 307.79,174.1 307.3,174.26
S$10503
  Bottom 0: 307.3,174.26 306.79,174.35
S$10504
  Bottom 0: 306.79,174.35 306.27,174.35
S$10505
  Bottom 0: 306.27,174.35 305.76,174.26
S$10506
  Bottom 0: 305.76,174.26 305.27,174.1
S$10507
  Bottom 0: 305.27,174.1 304.82,173.85
S$10508
  Bottom 0: 304.82,173.85 304.41,173.53
S$10509
  Bottom 0: 304.41,173.53 304.06,173.15
S$10510
  Bottom 0: 304.06,173.15 303.77,172.72
S$10511
  Bottom 0: 303.77,172.72 303.57,172.24
S$10512
  Bottom 0: 303.57,172.24 303.44,171.75
S$10513
  Bottom 0: 303.44,171.75 303.4,171.23
S$10514
  Bottom 0: 303.4,171.23 303.44,170.71
S$10515
  Bottom 0: 303.44,170.71 303.57,170.21
S$10516
  Bottom 0: 303.57,170.21 303.77,169.73
S$10517
  Bottom 0: 303.77,169.73 304.06,169.3
S$10518
  Bottom 0: 304.06,169.3 304.41,168.92
S$10519
  Bottom 0: 304.41,168.92 304.82,168.6
S$10520
  Bottom 0: 304.82,168.6 305.27,168.36
S$10521
  Bottom 0: 305.27,168.36 305.76,168.19
S$10522
  Bottom 0: 305.76,168.19 306.27,168.1
S$10523
  Bottom 0: 289.52,169.5 289.82,169.57
S$10524
  Bottom 0: 289.82,169.57 290.08,169.72
S$10525
  Bottom 0: 290.08,169.72 290.28,169.94
S$10526
  Bottom 0: 290.28,169.94 290.42,170.22
S$10527
  Bottom 0: 290.42,170.22 290.46,170.51
S$10528
  Bottom 0: 290.46,170.51 290.42,170.81
S$10529
  Bottom 0: 290.42,170.81 290.28,171.09
S$10530
  Bottom 0: 290.28,171.09 290.08,171.31
S$10531
  Bottom 0: 290.08,171.31 289.82,171.46
S$10532
  Bottom 0: 289.82,171.46 289.52,171.53
S$10533
  Bottom 0: 289.52,171.53 289.22,171.51
S$10534
  Bottom 0: 289.22,171.51 288.94,171.39
S$10535
  Bottom 0: 288.94,171.39 288.7,171.21
S$10536
  Bottom 0: 288.7,171.21 288.53,170.96
S$10537
  Bottom 0: 288.53,170.96 288.44,170.67
S$10538
  Bottom 0: 288.44,170.67 288.44,170.36
S$10539
  Bottom 0: 288.44,170.36 288.53,170.07
S$10540
  Bottom 0: 288.53,170.07 288.7,169.82
S$10541
  Bottom 0: 288.7,169.82 288.94,169.64
S$10542
  Bottom 0: 288.94,169.64 289.22,169.53
S$10543
  Bottom 0: 289.22,169.53 289.52,169.5
S$10544
  Bottom 0: 287.2,172.48 287.2,172.97
S$10545
  Bottom 0: 287.2,172.97 286.71,172.97
S$10546
  Bottom 0: 286.71,172.97 286.75,172.87
S$10547
  Bottom 0: 286.75,172.87 286.92,172.64
S$10548
  Bottom 0: 286.92,172.64 287.16,172.49
S$10549
  Bottom 0: 287.16,172.49 287.2,172.48
S$10550
  Bottom 0: 287.8,172.49 287.97,172.56
S$10551
  Bottom 0: 287.97,172.56 288.18,172.75
S$10552
  Bottom 0: 288.18,172.75 288.3,172.97
S$10553
  Bottom 0: 288.3,172.97 287.8,172.97
S$10554
  Bottom 0: 287.8,172.97 287.8,172.49
S$10555
  Bottom 0: 287.8,173.57 288.3,173.57
S$10556
  Bottom 0: 288.3,173.57 288.18,173.8
S$10557
  Bottom 0: 288.18,173.8 287.97,173.99
S$10558
  Bottom 0: 287.97,173.99 287.8,174.06
S$10559
  Bottom 0: 287.8,174.06 287.8,173.57
S$10560
  Bottom 0: 288.99,177.1 288.99,177.81
S$10561
  Bottom 0: 288.99,177.81 288.29,177.81
S$10562
  Bottom 0: 288.29,177.81 288.43,177.56
S$10563
  Bottom 0: 288.43,177.56 288.67,177.3
S$10564
  Bottom 0: 288.67,177.3 288.96,177.11
S$10565
  Bottom 0: 288.96,177.11 288.99,177.1
S$10566
  Bottom 0: 290.13,177.11 290.31,177.19
S$10567
  Bottom 0: 290.31,177.19 290.58,177.42
S$10568
  Bottom 0: 290.58,177.42 290.79,177.7
S$10569
  Bottom 0: 290.79,177.7 290.83,177.81
S$10570
  Bottom 0: 290.83,177.81 290.13,177.81
S$10571
  Bottom 0: 290.13,177.81 290.13,177.11
S$10572
  Bottom 0: 59.64,102.36 59.66,102.49
S$10573
  Bottom 0: 59.66,102.49 59.61,102.81
S$10574
  Bottom 0: 59.61,102.81 59.47,103.11
S$10575
  Bottom 0: 59.47,103.11 59.26,103.35
S$10576
  Bottom 0: 59.26,103.35 58.99,103.53
S$10577
  Bottom 0: 58.99,103.53 58.68,103.62
S$10578
  Bottom 0: 58.68,103.62 58.35,103.62
S$10579
  Bottom 0: 58.35,103.62 58.23,103.58
S$10580
  Bottom 0: 58.23,103.58 56.25,105.56
S$10581
  Bottom 0: 56.25,105.56 56.25,117.24
S$10582
  Bottom 0: 56.25,117.24 56.24,117.33
S$10583
  Bottom 0: 56.24,117.33 56.22,117.41
S$10584
  Bottom 0: 56.22,117.41 56.19,117.5
S$10585
  Bottom 0: 56.19,117.5 56.14,117.57
S$10586
  Bottom 0: 56.14,117.57 56.08,117.64
S$10587
  Bottom 0: 56.08,117.64 52.47,121.24
S$10588
  Bottom 0: 52.47,121.24 52.51,121.54
S$10589
  Bottom 0: 52.51,121.54 52.46,121.86
S$10590
  Bottom 0: 52.46,121.86 52.33,122.16
S$10591
  Bottom 0: 52.33,122.16 52.11,122.4
S$10592
  Bottom 0: 52.11,122.4 51.84,122.58
S$10593
  Bottom 0: 51.84,122.58 51.53,122.67
S$10594
  Bottom 0: 51.53,122.67 51.21,122.67
S$10595
  Bottom 0: 51.21,122.67 50.9,122.58
S$10596
  Bottom 0: 50.9,122.58 50.62,122.4
S$10597
  Bottom 0: 50.62,122.4 50.41,122.16
S$10598
  Bottom 0: 50.41,122.16 50.27,121.86
S$10599
  Bottom 0: 50.27,121.86 50.23,121.54
S$10600
  Bottom 0: 50.23,121.54 50.27,121.22
S$10601
  Bottom 0: 50.27,121.22 50.41,120.92
S$10602
  Bottom 0: 50.41,120.92 50.62,120.67
S$10603
  Bottom 0: 50.62,120.67 50.9,120.5
S$10604
  Bottom 0: 50.9,120.5 51.21,120.41
S$10605
  Bottom 0: 51.21,120.41 51.53,120.41
S$10606
  Bottom 0: 51.53,120.41 51.66,120.45
S$10607
  Bottom 0: 51.66,120.45 55.11,117
S$10608
  Bottom 0: 55.11,117 55.11,114.62
S$10609
  Bottom 0: 55.11,114.62 54.92,114.87
S$10610
  Bottom 0: 54.92,114.87 54.65,115.1
S$10611
  Bottom 0: 54.65,115.1 54.35,115.25
S$10612
  Bottom 0: 54.35,115.25 54.35,116.06
S$10613
  Bottom 0: 54.35,116.06 54.35,116.13
S$10614
  Bottom 0: 54.35,116.13 54.33,116.19
S$10615
  Bottom 0: 54.33,116.19 54.3,116.26
S$10616
  Bottom 0: 54.3,116.26 54.27,116.32
S$10617
  Bottom 0: 54.27,116.32 54.22,116.37
S$10618
  Bottom 0: 54.22,116.37 50.49,120.11
S$10619
  Bottom 0: 50.49,120.11 50.43,120.15
S$10620
  Bottom 0: 50.43,120.15 50.37,120.19
S$10621
  Bottom 0: 50.37,120.19 50.31,120.21
S$10622
  Bottom 0: 50.31,120.21 50.25,120.23
S$10623
  Bottom 0: 50.25,120.23 50.17,120.23
S$10624
  Bottom 0: 50.17,120.23 46.62,120.23
S$10625
  Bottom 0: 46.62,120.23 37.79,129.06
S$10626
  Bottom 0: 37.79,129.06 38.12,129.04
S$10627
  Bottom 0: 38.12,129.04 38.47,129.1
S$10628
  Bottom 0: 38.47,129.1 38.78,129.25
S$10629
  Bottom 0: 38.78,129.25 39.05,129.47
S$10630
  Bottom 0: 39.05,129.47 39.26,129.76
S$10631
  Bottom 0: 39.26,129.76 39.38,130.08
S$10632
  Bottom 0: 39.38,130.08 39.43,130.43
S$10633
  Bottom 0: 39.43,130.43 39.38,130.77
S$10634
  Bottom 0: 39.38,130.77 39.26,131.1
S$10635
  Bottom 0: 39.26,131.1 39.05,131.38
S$10636
  Bottom 0: 39.05,131.38 38.78,131.61
S$10637
  Bottom 0: 38.78,131.61 38.47,131.76
S$10638
  Bottom 0: 38.47,131.76 38.12,131.82
S$10639
  Bottom 0: 38.12,131.82 37.77,131.8
S$10640
  Bottom 0: 37.77,131.8 37.44,131.69
S$10641
  Bottom 0: 37.44,131.69 37.15,131.51
S$10642
  Bottom 0: 37.15,131.51 36.96,131.31
S$10643
  Bottom 0: 36.96,131.31 36.96,134.71
S$10644
  Bottom 0: 36.96,134.71 38.39,136.14
S$10645
  Bottom 0: 38.39,136.14 38.33,135.96
S$10646
  Bottom 0: 38.33,135.96 38.29,135.51
S$10647
  Bottom 0: 38.29,135.51 38.33,135.06
S$10648
  Bottom 0: 38.33,135.06 38.46,134.63
S$10649
  Bottom 0: 38.46,134.63 38.67,134.24
S$10650
  Bottom 0: 38.67,134.24 38.96,133.89
S$10651
  Bottom 0: 38.96,133.89 39.3,133.61
S$10652
  Bottom 0: 39.3,133.61 39.7,133.4
S$10653
  Bottom 0: 39.7,133.4 40.13,133.27
S$10654
  Bottom 0: 40.13,133.27 40.57,133.22
S$10655
  Bottom 0: 40.57,133.22 41.02,133.27
S$10656
  Bottom 0: 41.02,133.27 41.45,133.4
S$10657
  Bottom 0: 41.45,133.4 41.84,133.61
S$10658
  Bottom 0: 41.84,133.61 42.19,133.89
S$10659
  Bottom 0: 42.19,133.89 42.47,134.24
S$10660
  Bottom 0: 42.47,134.24 42.69,134.63
S$10661
  Bottom 0: 42.69,134.63 42.81,135.06
S$10662
  Bottom 0: 42.81,135.06 42.86,135.51
S$10663
  Bottom 0: 42.86,135.51 42.81,135.96
S$10664
  Bottom 0: 42.81,135.96 42.69,136.38
S$10665
  Bottom 0: 42.69,136.38 42.47,136.78
S$10666
  Bottom 0: 42.47,136.78 42.19,137.12
S$10667
  Bottom 0: 42.19,137.12 41.84,137.41
S$10668
  Bottom 0: 41.84,137.41 41.45,137.62
S$10669
  Bottom 0: 41.45,137.62 41.02,137.75
S$10670
  Bottom 0: 41.02,137.75 40.57,137.79
S$10671
  Bottom 0: 40.57,137.79 40.13,137.75
S$10672
  Bottom 0: 40.13,137.75 39.94,137.69
S$10673
  Bottom 0: 39.94,137.69 40.89,138.65
S$10674
  Bottom 0: 40.89,138.65 40.93,138.7
S$10675
  Bottom 0: 40.93,138.7 40.98,138.76
S$10676
  Bottom 0: 40.98,138.76 41,138.82
S$10677
  Bottom 0: 41,138.82 41.02,138.88
S$10678
  Bottom 0: 41.02,138.88 41.02,138.96
S$10679
  Bottom 0: 41.02,138.96 41.02,139.81
S$10680
  Bottom 0: 41.02,139.81 41.09,139.72
S$10681
  Bottom 0: 41.09,139.72 41.37,139.55
S$10682
  Bottom 0: 41.37,139.55 41.68,139.46
S$10683
  Bottom 0: 41.68,139.46 42.01,139.46
S$10684
  Bottom 0: 42.01,139.46 42.32,139.55
S$10685
  Bottom 0: 42.32,139.55 42.59,139.72
S$10686
  Bottom 0: 42.59,139.72 42.8,139.97
S$10687
  Bottom 0: 42.8,139.97 42.94,140.27
S$10688
  Bottom 0: 42.94,140.27 42.99,140.59
S$10689
  Bottom 0: 42.99,140.59 42.94,140.91
S$10690
  Bottom 0: 42.94,140.91 42.8,141.21
S$10691
  Bottom 0: 42.8,141.21 42.59,141.45
S$10692
  Bottom 0: 42.59,141.45 42.32,141.63
S$10693
  Bottom 0: 42.32,141.63 42.01,141.72
S$10694
  Bottom 0: 42.01,141.72 41.68,141.72
S$10695
  Bottom 0: 41.68,141.72 41.37,141.63
S$10696
  Bottom 0: 41.37,141.63 41.09,141.45
S$10697
  Bottom 0: 41.09,141.45 41.02,141.36
S$10698
  Bottom 0: 41.02,141.36 41.02,143.57
S$10699
  Bottom 0: 41.02,143.57 41.17,143.72
S$10700
  Bottom 0: 41.17,143.72 41.18,143.72
S$10701
  Bottom 0: 41.18,143.72 43.15,145.69
S$10702
  Bottom 0: 43.15,145.69 45.41,145.69
S$10703
  Bottom 0: 45.41,145.69 44.7,144.99
S$10704
  Bottom 0: 44.7,144.99 44.63,145.01
S$10705
  Bottom 0: 44.63,145.01 44.31,145.03
S$10706
  Bottom 0: 44.31,145.03 43.98,144.97
S$10707
  Bottom 0: 43.98,144.97 43.7,144.82
S$10708
  Bottom 0: 43.7,144.82 43.46,144.6
S$10709
  Bottom 0: 43.46,144.6 43.29,144.32
S$10710
  Bottom 0: 43.29,144.32 43.2,144.01
S$10711
  Bottom 0: 43.2,144.01 43.2,143.68
S$10712
  Bottom 0: 43.2,143.68 43.29,143.37
S$10713
  Bottom 0: 43.29,143.37 43.46,143.09
S$10714
  Bottom 0: 43.46,143.09 43.7,142.87
S$10715
  Bottom 0: 43.7,142.87 43.98,142.72
S$10716
  Bottom 0: 43.98,142.72 44.31,142.66
S$10717
  Bottom 0: 44.31,142.66 44.63,142.68
S$10718
  Bottom 0: 44.63,142.68 44.94,142.78
S$10719
  Bottom 0: 44.94,142.78 45.2,142.97
S$10720
  Bottom 0: 45.2,142.97 45.41,143.23
S$10721
  Bottom 0: 45.41,143.23 45.53,143.52
S$10722
  Bottom 0: 45.53,143.52 45.58,143.84
S$10723
  Bottom 0: 45.58,143.84 45.56,143.94
S$10724
  Bottom 0: 45.56,143.94 45.7,143.8
S$10725
  Bottom 0: 45.7,143.8 45.7,141.57
S$10726
  Bottom 0: 45.7,141.57 45.7,141.5
S$10727
  Bottom 0: 45.7,141.5 45.72,141.44
S$10728
  Bottom 0: 45.72,141.44 45.74,141.38
S$10729
  Bottom 0: 45.74,141.38 45.79,141.31
S$10730
  Bottom 0: 45.79,141.31 45.82,141.26
S$10731
  Bottom 0: 45.82,141.26 54.43,132.65
S$10732
  Bottom 0: 54.43,132.65 54.49,132.61
S$10733
  Bottom 0: 54.49,132.61 54.55,132.57
S$10734
  Bottom 0: 54.55,132.57 54.61,132.54
S$10735
  Bottom 0: 54.61,132.54 54.68,132.53
S$10736
  Bottom 0: 54.68,132.53 54.74,132.53
S$10737
  Bottom 0: 54.74,132.53 62.12,132.53
S$10738
  Bottom 0: 62.12,132.53 62.14,132.46
S$10739
  Bottom 0: 62.14,132.46 62.31,132.15
S$10740
  Bottom 0: 62.31,132.15 62.55,131.89
S$10741
  Bottom 0: 62.55,131.89 62.84,131.7
S$10742
  Bottom 0: 62.84,131.7 63.17,131.6
S$10743
  Bottom 0: 63.17,131.6 63.52,131.58
S$10744
  Bottom 0: 63.52,131.58 63.87,131.64
S$10745
  Bottom 0: 63.87,131.64 64.19,131.79
S$10746
  Bottom 0: 64.19,131.79 64.45,132.01
S$10747
  Bottom 0: 64.45,132.01 64.66,132.3
S$10748
  Bottom 0: 64.66,132.3 64.79,132.62
S$10749
  Bottom 0: 64.79,132.62 64.84,132.97
S$10750
  Bottom 0: 64.84,132.97 64.79,133.31
S$10751
  Bottom 0: 64.79,133.31 64.66,133.64
S$10752
  Bottom 0: 64.66,133.64 64.45,133.92
S$10753
  Bottom 0: 64.45,133.92 64.19,134.15
S$10754
  Bottom 0: 64.19,134.15 63.87,134.3
S$10755
  Bottom 0: 63.87,134.3 63.52,134.36
S$10756
  Bottom 0: 63.52,134.36 63.17,134.34
S$10757
  Bottom 0: 63.17,134.34 62.84,134.23
S$10758
  Bottom 0: 62.84,134.23 62.55,134.05
S$10759
  Bottom 0: 62.55,134.05 62.31,133.79
S$10760
  Bottom 0: 62.31,133.79 62.14,133.48
S$10761
  Bottom 0: 62.14,133.48 62.12,133.41
S$10762
  Bottom 0: 62.12,133.41 60.53,133.41
S$10763
  Bottom 0: 60.53,133.41 60.9,133.61
S$10764
  Bottom 0: 60.9,133.61 61.24,133.89
S$10765
  Bottom 0: 61.24,133.89 61.53,134.24
S$10766
  Bottom 0: 61.53,134.24 61.74,134.63
S$10767
  Bottom 0: 61.74,134.63 61.87,135.06
S$10768
  Bottom 0: 61.87,135.06 61.91,135.51
S$10769
  Bottom 0: 61.91,135.51 61.87,135.96
S$10770
  Bottom 0: 61.87,135.96 61.74,136.38
S$10771
  Bottom 0: 61.74,136.38 61.53,136.78
S$10772
  Bottom 0: 61.53,136.78 61.24,137.12
S$10773
  Bottom 0: 61.24,137.12 60.9,137.41
S$10774
  Bottom 0: 60.9,137.41 60.5,137.62
S$10775
  Bottom 0: 60.5,137.62 60.08,137.75
S$10776
  Bottom 0: 60.08,137.75 59.63,137.79
S$10777
  Bottom 0: 59.63,137.79 59.18,137.75
S$10778
  Bottom 0: 59.18,137.75 58.76,137.62
S$10779
  Bottom 0: 58.76,137.62 58.36,137.41
S$10780
  Bottom 0: 58.36,137.41 58.01,137.12
S$10781
  Bottom 0: 58.01,137.12 57.73,136.78
S$10782
  Bottom 0: 57.73,136.78 57.52,136.38
S$10783
  Bottom 0: 57.52,136.38 57.39,135.96
S$10784
  Bottom 0: 57.39,135.96 57.34,135.51
S$10785
  Bottom 0: 57.34,135.51 57.39,135.06
S$10786
  Bottom 0: 57.39,135.06 57.52,134.63
S$10787
  Bottom 0: 57.52,134.63 57.73,134.24
S$10788
  Bottom 0: 57.73,134.24 58.01,133.89
S$10789
  Bottom 0: 58.01,133.89 58.36,133.61
S$10790
  Bottom 0: 58.36,133.61 58.73,133.41
S$10791
  Bottom 0: 58.73,133.41 54.93,133.41
S$10792
  Bottom 0: 54.93,133.41 49.72,138.62
S$10793
  Bottom 0: 49.72,138.62 49.88,138.56
S$10794
  Bottom 0: 49.88,138.56 50.18,138.54
S$10795
  Bottom 0: 50.18,138.54 50.48,138.61
S$10796
  Bottom 0: 50.48,138.61 50.74,138.76
S$10797
  Bottom 0: 50.74,138.76 50.77,138.8
S$10798
  Bottom 0: 50.77,138.8 68.48,138.8
S$10799
  Bottom 0: 68.48,138.8 68.65,138.67
S$10800
  Bottom 0: 68.65,138.67 68.92,138.56
S$10801
  Bottom 0: 68.92,138.56 69.23,138.54
S$10802
  Bottom 0: 69.23,138.54 69.53,138.61
S$10803
  Bottom 0: 69.53,138.61 69.79,138.76
S$10804
  Bottom 0: 69.79,138.76 69.99,138.98
S$10805
  Bottom 0: 69.99,138.98 70.12,139.25
S$10806
  Bottom 0: 70.12,139.25 70.17,139.52
S$10807
  Bottom 0: 70.17,139.52 78.09,131.59
S$10808
  Bottom 0: 78.09,131.59 78.09,130.72
S$10809
  Bottom 0: 78.09,130.72 77.49,130.12
S$10810
  Bottom 0: 77.49,130.12 77.53,130.43
S$10811
  Bottom 0: 77.53,130.43 77.48,130.77
S$10812
  Bottom 0: 77.48,130.77 77.36,131.1
S$10813
  Bottom 0: 77.36,131.1 77.15,131.38
S$10814
  Bottom 0: 77.15,131.38 76.88,131.61
S$10815
  Bottom 0: 76.88,131.61 76.57,131.76
S$10816
  Bottom 0: 76.57,131.76 76.22,131.82
S$10817
  Bottom 0: 76.22,131.82 75.87,131.8
S$10818
  Bottom 0: 75.87,131.8 75.54,131.69
S$10819
  Bottom 0: 75.54,131.69 75.51,131.68
S$10820
  Bottom 0: 75.51,131.68 74.94,132.25
S$10821
  Bottom 0: 74.94,132.25 74.89,132.29
S$10822
  Bottom 0: 74.89,132.29 74.83,132.33
S$10823
  Bottom 0: 74.83,132.33 74.77,132.35
S$10824
  Bottom 0: 74.77,132.35 74.7,132.37
S$10825
  Bottom 0: 74.7,132.37 74.63,132.38
S$10826
  Bottom 0: 74.63,132.38 70.06,132.38
S$10827
  Bottom 0: 70.06,132.38 69.99,132.51
S$10828
  Bottom 0: 69.99,132.51 69.79,132.72
S$10829
  Bottom 0: 69.79,132.72 69.53,132.88
S$10830
  Bottom 0: 69.53,132.88 69.23,132.94
S$10831
  Bottom 0: 69.23,132.94 68.92,132.92
S$10832
  Bottom 0: 68.92,132.92 68.65,132.81
S$10833
  Bottom 0: 68.65,132.81 68.41,132.62
S$10834
  Bottom 0: 68.41,132.62 68.24,132.38
S$10835
  Bottom 0: 68.24,132.38 68.15,132.09
S$10836
  Bottom 0: 68.15,132.09 68.15,131.78
S$10837
  Bottom 0: 68.15,131.78 68.24,131.49
S$10838
  Bottom 0: 68.24,131.49 68.41,131.24
S$10839
  Bottom 0: 68.41,131.24 68.65,131.05
S$10840
  Bottom 0: 68.65,131.05 68.92,130.94
S$10841
  Bottom 0: 68.92,130.94 69.23,130.92
S$10842
  Bottom 0: 69.23,130.92 69.53,130.99
S$10843
  Bottom 0: 69.53,130.99 69.79,131.14
S$10844
  Bottom 0: 69.79,131.14 69.99,131.36
S$10845
  Bottom 0: 69.99,131.36 70.06,131.49
S$10846
  Bottom 0: 70.06,131.49 74.44,131.49
S$10847
  Bottom 0: 74.44,131.49 74.89,131.04
S$10848
  Bottom 0: 74.89,131.04 74.83,130.94
S$10849
  Bottom 0: 74.83,130.94 74.75,130.6
S$10850
  Bottom 0: 74.75,130.6 74.75,130.25
S$10851
  Bottom 0: 74.75,130.25 74.83,129.92
S$10852
  Bottom 0: 74.83,129.92 75,129.61
S$10853
  Bottom 0: 75,129.61 75.25,129.35
S$10854
  Bottom 0: 75.25,129.35 75.54,129.16
S$10855
  Bottom 0: 75.54,129.16 75.87,129.06
S$10856
  Bottom 0: 75.87,129.06 76.22,129.04
S$10857
  Bottom 0: 76.22,129.04 76.45,129.08
S$10858
  Bottom 0: 76.45,129.08 73.3,125.93
S$10859
  Bottom 0: 73.3,125.93 73.21,125.96
S$10860
  Bottom 0: 73.21,125.96 72.89,125.98
S$10861
  Bottom 0: 72.89,125.98 72.57,125.91
S$10862
  Bottom 0: 72.57,125.91 72.28,125.77
S$10863
  Bottom 0: 72.28,125.77 72.05,125.54
S$10864
  Bottom 0: 72.05,125.54 71.87,125.27
S$10865
  Bottom 0: 71.87,125.27 71.78,124.95
S$10866
  Bottom 0: 71.78,124.95 71.78,124.63
S$10867
  Bottom 0: 71.78,124.63 71.87,124.31
S$10868
  Bottom 0: 71.87,124.31 72.05,124.04
S$10869
  Bottom 0: 72.05,124.04 72.28,123.81
S$10870
  Bottom 0: 72.28,123.81 72.57,123.67
S$10871
  Bottom 0: 72.57,123.67 72.89,123.6
S$10872
  Bottom 0: 72.89,123.6 73.21,123.62
S$10873
  Bottom 0: 73.21,123.62 73.52,123.73
S$10874
  Bottom 0: 73.52,123.73 73.78,123.92
S$10875
  Bottom 0: 73.78,123.92 73.99,124.17
S$10876
  Bottom 0: 73.99,124.17 74.11,124.47
S$10877
  Bottom 0: 74.11,124.47 74.16,124.79
S$10878
  Bottom 0: 74.16,124.79 74.11,125.11
S$10879
  Bottom 0: 74.11,125.11 74.11,125.13
S$10880
  Bottom 0: 74.11,125.13 79.06,130.09
S$10881
  Bottom 0: 79.06,130.09 79.13,130.16
S$10882
  Bottom 0: 79.13,130.16 79.17,130.23
S$10883
  Bottom 0: 79.17,130.23 79.21,130.31
S$10884
  Bottom 0: 79.21,130.31 79.22,130.4
S$10885
  Bottom 0: 79.22,130.4 79.23,130.49
S$10886
  Bottom 0: 79.23,130.49 79.23,131.36
S$10887
  Bottom 0: 79.23,131.36 79.24,131.36
S$10888
  Bottom 0: 79.24,131.36 79.31,131.43
S$10889
  Bottom 0: 79.31,131.43 81.12,133.24
S$10890
  Bottom 0: 81.12,133.24 81.09,133.14
S$10891
  Bottom 0: 81.09,133.14 81.09,132.79
S$10892
  Bottom 0: 81.09,132.79 81.18,132.46
S$10893
  Bottom 0: 81.18,132.46 81.35,132.15
S$10894
  Bottom 0: 81.35,132.15 81.59,131.89
S$10895
  Bottom 0: 81.59,131.89 81.89,131.7
S$10896
  Bottom 0: 81.89,131.7 82.22,131.6
S$10897
  Bottom 0: 82.22,131.6 82.57,131.58
S$10898
  Bottom 0: 82.57,131.58 82.92,131.64
S$10899
  Bottom 0: 82.92,131.64 83.23,131.79
S$10900
  Bottom 0: 83.23,131.79 83.5,132.01
S$10901
  Bottom 0: 83.5,132.01 83.71,132.3
S$10902
  Bottom 0: 83.71,132.3 83.83,132.62
S$10903
  Bottom 0: 83.83,132.62 83.88,132.97
S$10904
  Bottom 0: 83.88,132.97 83.83,133.31
S$10905
  Bottom 0: 83.83,133.31 83.73,133.58
S$10906
  Bottom 0: 83.73,133.58 84.16,134.01
S$10907
  Bottom 0: 84.16,134.01 84.2,134.06
S$10908
  Bottom 0: 84.2,134.06 84.24,134.12
S$10909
